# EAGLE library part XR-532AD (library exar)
PULSE DETECTOR
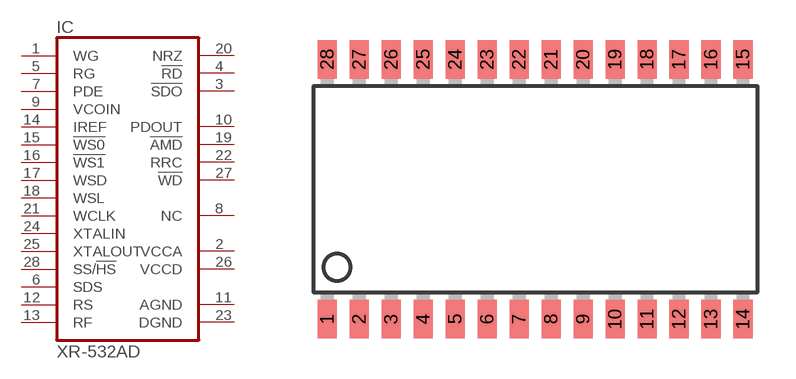
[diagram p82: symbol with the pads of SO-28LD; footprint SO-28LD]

Designator prefix IC

## XR-532AD (OC_FARNELL: unknown; OC_NEWARK: unknown)  [SO-28LD]
1  WG  in
2  VCCA  pwr
3  !SDO
4  !RD
5  RG  in
6  SDS  in
7  PDE  in
8  NC  out
9  VCOIN  in
10  PDOUT  out
11  AGND  pwr
12  RS  in
13  RF  in
14  IREF  in
15  !WS0  in
16  !WS1  in
17  WSD  in
18  WSL  in
19  !AMD  out
20  NRZ
21  WCLK  in
22  RRC  out
23  DGND  pwr
24  XTALIN  in
25  XTALOUT  in
26  VCCD  pwr
27  !WD  out
28  SS/!HS  in

## Footprint SO-28LD (pad centres in mm)
Small Outline Package
smd 0.762 x 1.524: 1 -8.255,-5.156; 2 -6.985,-5.156; 3 -5.715,-5.156; 4 -4.445,-5.156; 5 -3.175,-5.156; 6 -1.905,-5.156; 7 -0.635,-5.156; 8 0.635,-5.156; 9 1.905,-5.156; 10 3.175,-5.156; 11 4.445,-5.156; 12 5.715,-5.156; 13 6.985,-5.156; 14 8.255,-5.156; 15 8.255,5.156; 16 6.985,5.156; 17 5.715,5.156; 18 4.445,5.156; 19 3.175,5.156; 20 1.905,5.156; 21 0.635,5.156; 22 -0.635,5.156; 23 -1.905,5.156; 24 -3.175,5.156; 25 -4.445,5.156; 26 -5.715,5.156; 27 -6.985,5.156; 28 -8.255,5.156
